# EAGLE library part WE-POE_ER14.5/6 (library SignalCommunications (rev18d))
Power over Ethernet Transformer Characteristics Flyback transformer designed for PoE PDs Input voltage: 36 V to 57 V Switching frequencies: 200–500 kHz Operating temperature: –40 ºC to +125 ºC Insulation test voltage: 1.5 kVAC/1 min Different output powers and voltages available Applications Suitable for PoE IC’s like LTC4267, TPS 23750, TPS 23770, LM5070, LM 5071, LM 5072 Details see: http://katalog.we-online.de/en/pbs/WE-PoE? Updated by Dan Xu 2014-07-08 2014 (C) Wurth Elektronik
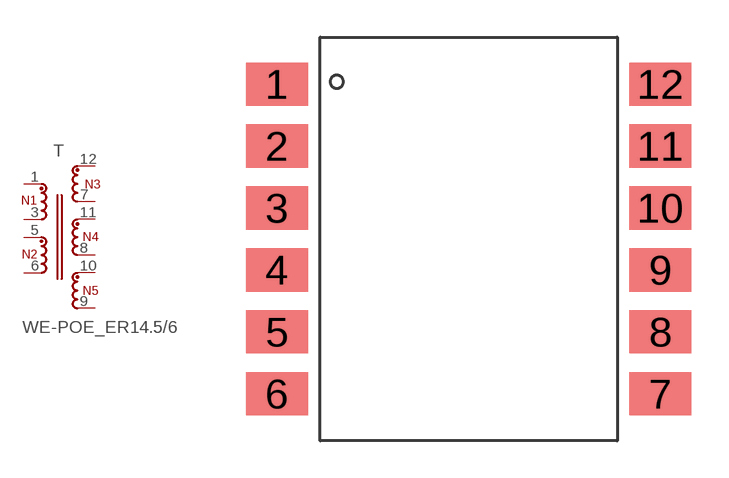
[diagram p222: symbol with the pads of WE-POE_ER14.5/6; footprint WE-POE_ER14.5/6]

Designator prefix T

## WE-POE_ER14.5/6_749119218, WE-POE_ER14.5/6_749119250  [WE-POE_ER14.5/6]
1  1  pas
3  2  pas
5  3  pas
6  4  pas
7  6  pas
8  8  pas
9  10  pas
10  9  pas
11  7  pas
12  5  pas

## Footprint WE-POE_ER14.5/6 (pad centres in mm)
Transformer, ER14.5/6 SMD 12Pin
smd 2.5 x 1.75: 1 -7.75,6.25; 2 -7.75,3.75; 3 -7.75,1.25; 4 -7.75,-1.25; 5 -7.75,-3.75; 6 -7.75,-6.25; 7 7.75,-6.25; 8 7.75,-3.75; 9 7.75,-1.25; 10 7.75,1.25; 11 7.75,3.75; 12 7.75,6.25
